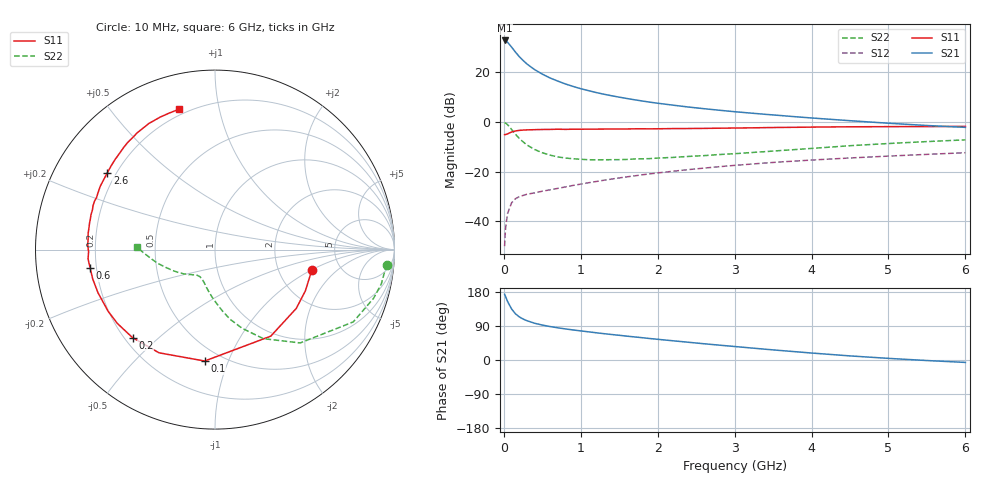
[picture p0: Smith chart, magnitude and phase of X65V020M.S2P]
! SIEMENS Small Signal Semiconductors
! BFP193W
! Si NPN RF Bipolar Junction Transistor in SOT343
! VCE = 5 V  IC = 20 mA
! Common Emitter S-Parameters:  April 1994
# GHz  S  MA  R  50
!  f  S11  S21  S12  S22
! GHz  MAG  ANG  MAG  ANG  MAG  ANG  MAG  ANG
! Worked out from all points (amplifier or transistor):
!   40 points, 10 MHz to 6 GHz, reference 50 ohm
!   highest |S21| = 32.6 dB at 10 MHz (marker M1)
!   |S21| within 3 dB of that: start of sweep to 109 MHz
!   unconditionally stable (mu >= 1): 980.2 MHz to 4.206 GHz
!   at 200 MHz: K = 0.34, MSG = 28.1 dB, |S12| = -30.1 dB
!   at 1.5 GHz: K = 1.10, MAG = 14.3 dB, |S12| = -22.5 dB
!   at 6 GHz: K = 0.94, MSG = 5.1 dB, |S12| = -12.4 dB
!   lowest NFmin = 1.40 dB at 450 MHz
!   S11 on the Smith chart (normalised r, x): 10 MHz: 3.08, -1.02; 100 MHz: 0.41, -0.83; 200 MHz: 0.23, -0.41; 600 MHz: 0.18, -0.07; 2.6 GHz: 0.17, +0.31; 6 GHz: 0.17, +0.76
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0.01  0.5513 -12.1  42.76 173.4  0.0032 89.2  0.9597 -5.0
0.02  0.5535 -24.5  42.51 168.8  0.0065 78.3  0.9461 -11.7
0.03  0.5589 -35.9  41.62 163.6  0.0093 78.1  0.924 -17.1
0.05  0.5737 -57.2  39.1 153.8  0.0146 67.7  0.8694 -27.6
0.1  0.6235 -95.3  31.55 134.9  0.0236 52.9  0.7042 -47.6
0.15  0.6542 -118.5  25.08 122.1  0.0286 45.3  0.5646 -61.5
0.2  0.6721 -133.1  20.3 113.9  0.0314 41.3  0.4646 -70.9
0.25  0.682 -142.9  16.99 108.1  0.0333 39.3  0.396 -77.9
0.3  0.6875 -150.1  14.43 103.7  0.0352 38.4  0.3426 -83.3
0.4  0.6949 -159.8  11.12 97.0  0.0375 38.8  0.278 -91.6
0.5  0.7006 -166.5  9.036 92.2  0.0405 40.3  0.2395 -97.9
0.6  0.703 -171.5  7.567 88.3  0.0432 42.5  0.2147 -103.0
0.8  0.7044 -179.0  5.736 82.0  0.0494 46.2  0.1877 -110.2
1.1  0.7125 172.8  4.216 74.3  0.0598 50.0  0.1733 -118.0
1.3  0.7143 168.2  3.571 69.5  0.0672 51.6  0.1731 -121.4
1.6  0.7175 162.1  2.929 62.9  0.0787 53.0  0.1759 -125.7
2.2  0.7301 151.2  2.154 50.7  0.1019 52.9  0.193 -134.2
2.6  0.737 144.5  1.831 42.9  0.1177 51.7  0.2093 -139.6
3.2  0.755 134.9  1.498 32.0  0.1411 48.8  0.2407 -148.0
4.5  0.7935 117.6  1.051 10.8  0.1879 41.0  0.3313 -167.0
5.5  0.802 108.8  0.842 -1.4  0.2219 35.1  0.4007 -177.7
6  0.8072 104.5  0.773 -6.4  0.2398 32.4  0.434 178.2
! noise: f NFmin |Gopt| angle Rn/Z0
0.45  1.4  0.3  160  0.1
0.9  1.45  0.34  172  0.11
1.8  2.2  0.56  -148  0.2
